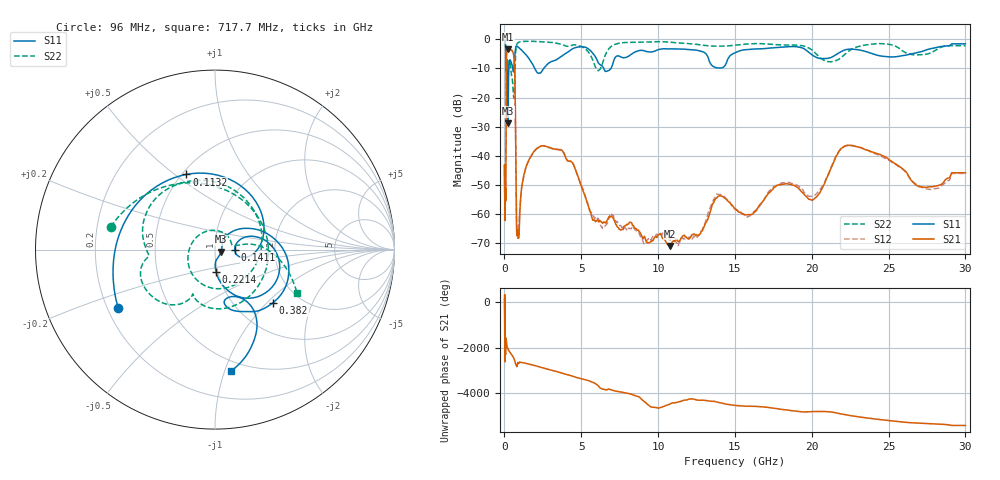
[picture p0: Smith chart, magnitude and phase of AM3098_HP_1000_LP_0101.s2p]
! Date/Time: Thu, Feb 28, 2019 8:39 AM
! Network Analyzer: Agilent Technologies E8364B Rev: A.07.50.67
! Sweep from 0.010 to 30.000 GHz, 1601 Points, Sweep Type: LOG
! Power Supply: 5.023 V, 0.002 A
# Hz S DB R 50
!freq MagS11 AngS11 MagS21 AngS21 MagS12 AngS12 MagS22 AngS22
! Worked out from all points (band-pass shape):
!   1601 points, 10 MHz to 30 GHz, reference 50 ohm
!   highest |S21| = -3.36 dB at 236.3 MHz (marker M1); lowest = -71.0 dB at 10.76 GHz (marker M2)
!   |S21| within 3 dB of the highest: 127.2 MHz to 622.5 MHz (495.3 MHz wide, 132 % of centre)
!   lowest |S11| = -28.9 dB at 236.3 MHz (marker M3), VSWR 1.07, Z = 53.5 - j1.32 ohm
!   |S11| at or under -10 dB: 198.6 MHz to 287.3 MHz (88.69 MHz wide, 36.5 % of centre); 1.975 GHz to 2.551 GHz (576.7 MHz wide, 25.5 % of centre); 6.465 GHz to 6.928 GHz (463.6 MHz wide, 6.92 % of centre)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
!   |S22| runs from -20.2 to -0.5 dB; largest |S21 - S12| = 0.0099
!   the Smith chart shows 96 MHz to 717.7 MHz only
!   S11 on the Smith chart (normalised r, x): 96 MHz: 0.24, -0.26; 113.2 MHz: 0.53, +0.55; 141.1 MHz: 1.25, -0.00; 221.4 MHz: 0.98, -0.24; 382 MHz: 1.48, -1.08; 717.7 MHz: 0.41, -1.05
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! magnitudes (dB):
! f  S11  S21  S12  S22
! 10 MHz  -0.4  -43.5  -43.9  -0.5
! 38.04 MHz  -0.5  -60.2  -59.8  -0.9
! 84.29 MHz  -2.4  -53.6  -54.8  -2.7
! 96 MHz  -4.0  -41.4  -42.1  -4.5
! 113.2 MHz  -7.0  -15.8  -15.8  -10.5
! 141.1 MHz  -19.2  -4.5  -4.5  -11.0
! 144.7 MHz  -18.5  -4.4  -4.3  -10.5
! 221.4 MHz  -18.2  -3.4  -3.4  -8.5
! 236.3 MHz  -28.9  -3.4  -3.3  -8.7
! 382 MHz  -7.2  -3.7  -3.6  -8.6
! 550.5 MHz  -10.5  -4.4  -4.4  -16.6
! 655.8 MHz  -7.1  -9.2  -9.2  -16.3
! 717.7 MHz  -3.3  -28.8  -28.6  -5.7
! 785.3 MHz  -2.3  -64.2  -62.1  -2.0
! 863.6 MHz  -2.5  -65.5  -67.9  -1.2
! 2.084 GHz  -11.1  -37.6  -37.8  -0.7
! 3.76 GHz  -5.6  -38.3  -38.3  -1.8
! 7.926 GHz  -6.2  -63.8  -65.3  -1.0
! 10.76 GHz  -3.3  -71.0  -68.9  -1.0
! 20.1 GHz  -5.6  -55.1  -54.0  -4.0
! 22.56 GHz  -3.4  -36.5  -36.5  -3.5
! 30 GHz  -1.5  -45.9  -46.1  -2.2
